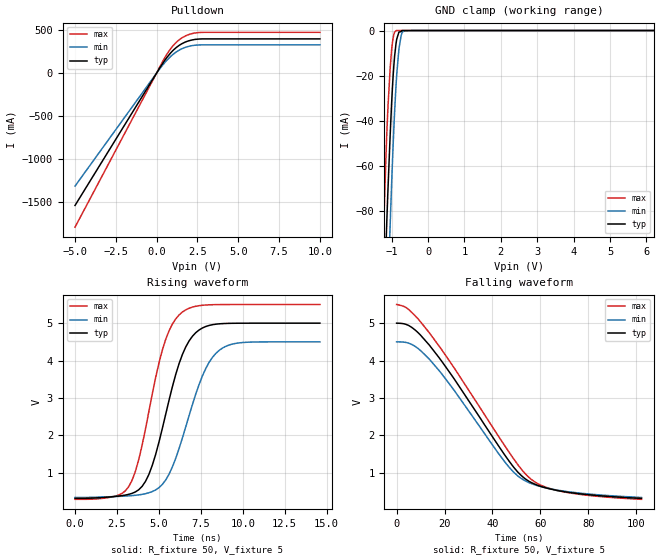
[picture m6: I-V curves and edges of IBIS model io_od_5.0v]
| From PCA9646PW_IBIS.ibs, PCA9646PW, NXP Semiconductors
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[Model]   io_od_5.0v
Model_type I/O_open_drain
Vinl=5.000E-01
Vinh=2.000E+00
Vref=5.000E+00
Rref=2.000E+03
Cref=0.000E+00
Vmeas=1.600E+00
C_comp   1.110E-12   1.080E-12   1.140E-12
[Voltage Range]   5.000E+00   4.500E+00   5.500E+00
[POWER Clamp Reference]   5.000E+00   4.500E+00   5.500E+00
[GND Clamp Reference]   0.000E+00   0.000E+00   0.000E+00
[Pullup Reference]   5.000E+00   4.500E+00   5.500E+00
[Pulldown Reference]   0.000E+00   0.000E+00   0.000E+00
[Temperature Range]   25   85   -40
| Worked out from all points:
|   slope of the pulldown table from 0 to 0.75 V, typ, clamps not added: 3.58 ohm
|   GND clamp passes 1 mA (typ) near -0.81 V on its own axis
|   rising waveform, R_fixture 50, V_fixture 5: 20-80 % time 1.68ns typ, 1.86ns min, 1.54ns max; typ from 0.31 V to 5 V
|   falling waveform, R_fixture 50, V_fixture 5: 20-80 % time 29.7ns typ, 28.1ns min, 32.4ns max; typ from 5 V to 0.31 V
[GND Clamp]
-5V       -2.067A    -2.236A    -1.848A
-1.2V     -119.7mA   -167.3mA   -77.77mA
-1.14V    -88.15mA   -134.1mA   -48.62mA
-1.1V     -70.15mA   -114.2mA   -33.65mA
-1.04V    -46.16mA   -86mA      -16.59mA
-1V       -32.06mA   -67.85mA   -8.494mA
-960mV    -20.41mA   -51.19mA   -3.37mA
-880mV    -5.786mA   -24.45mA   -65.51uA
-800mV    -695.4uA   -8.192mA   0A
-740mV    -503uA     -2.25mA    0A
-680mV    0A         -216.6uA   0A
10V       0A         0A         0A
[Pulldown]
-5V       -1.538A    -1.313A    -1.79A
380mV     114.1mA    94.13mA    138mA
860mV     233.7mA    192.7mA    282.5mA
1.38V     321.3mA    265.7mA    385.8mA
1.94V     372.5mA    308.7mA    444.9mA
2.68V     395.5mA    326.8mA    471.4mA
10V       396.5mA    327.3mA    472.7mA
[Rising Waveform]
R_fixture = 50
V_fixture = 5
V_fixture_min = 4.5
V_fixture_max = 5.5
0s        310.4mV    334mV      284.8mV
2.4ns     362.5mV    359.6mV    369.5mV
3.2ns     418mV      377.6mV    623.5mV
3.8ns     542.1mV    403.7mV    1.351V
4.4ns     947.6mV    460mV      2.628V
5.4ns     2.55V      798mV      4.559V
6.4ns     4.16V      1.925V     5.298V
7.6ns     4.873V     3.595V     5.479V
8.6ns     4.983V     4.274V     5.498V
14.6ns    5V         4.5V       5.5V
[Falling Waveform]
R_fixture = 50
V_fixture = 5
V_fixture_min = 4.5
V_fixture_max = 5.5
0s        5V         4.5V       5.5V
6ns       4.901V     4.441V     5.308V
13.4ns    4.432V     4.053V     4.763V
23ns      3.604V     3.291V     3.9V
46.8ns    1.32V      1.155V     1.559V
52.2ns    911mV      835.6mV    1.079V
56.2ns    734.3mV    707.2mV    818.8mV
62.2ns    592.7mV    593.2mV    611.5mV
71.4ns    475.2mV    489.1mV    465.1mV
102.2ns   310.4mV    334mV      284.8mV
[Ramp]
dV/dt_r   2.8138E+00/1.6700E-09   2.4996E+00/1.8510E-09   3.1291E+00/1.5370E-09
dV/dt_f   2.8138E+00/2.9725E-08   2.4996E+00/2.8114E-08   3.1291E+00/3.2355E-08
R_load = 50
